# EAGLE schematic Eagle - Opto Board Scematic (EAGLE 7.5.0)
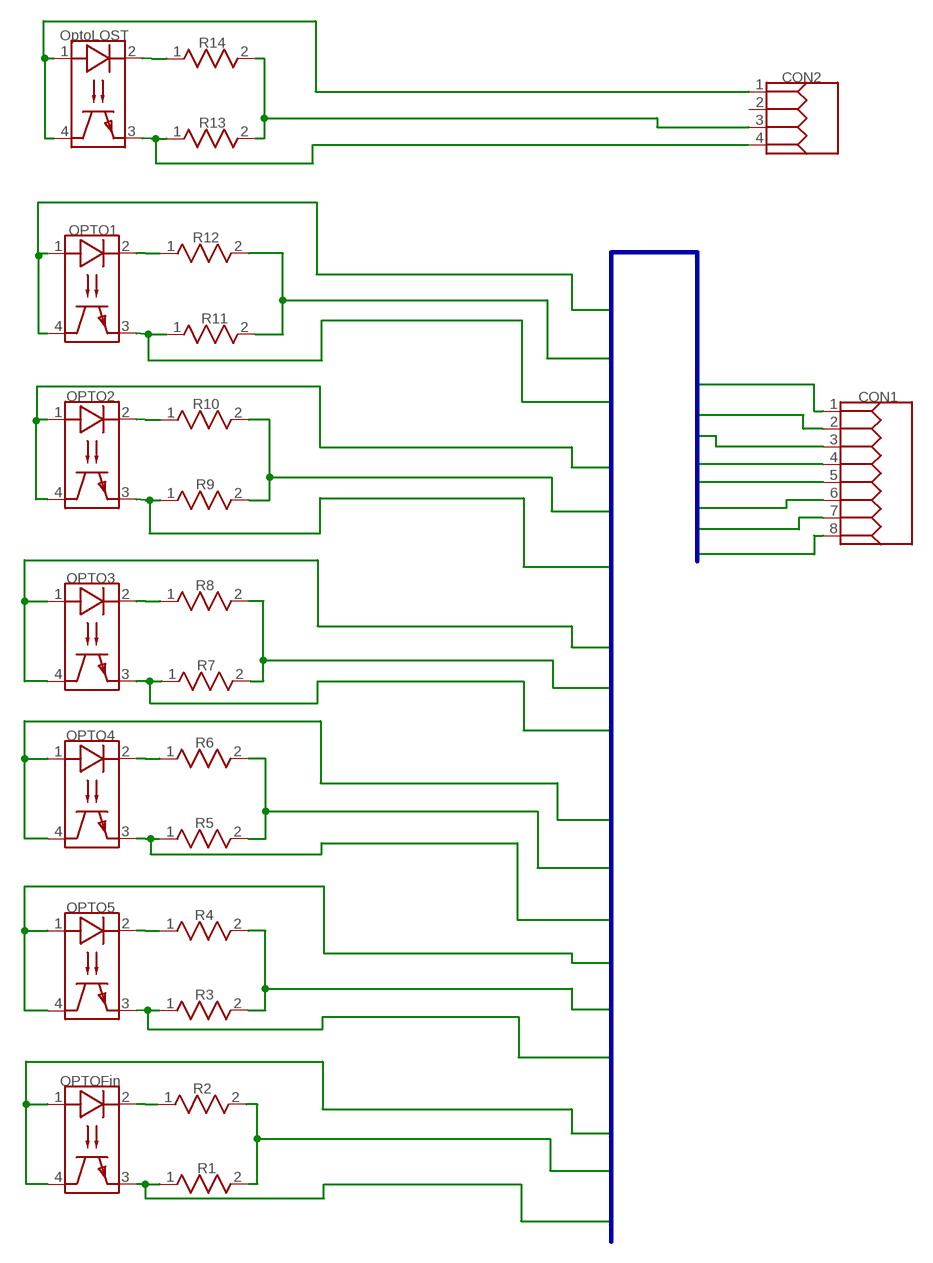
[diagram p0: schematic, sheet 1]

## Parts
CON1  51022-0800  [51022-0800]
CON2  51022-0400  [51022-0400]
OPTO1  TCRT1000  [TCRT1000]
OPTO2  TCRT1000  [TCRT1000]
OPTO3  TCRT1000  [TCRT1000]
OPTO4  TCRT1000  [TCRT1000]
OPTO5  TCRT1000  [TCRT1000]
OPTOFin  TCRT1000  [TCRT1000]
OptoLOST  TCRT1000  [TCRT1000]
R1  10K  RES  [RES_1206]
R2  150R  RES  [RES_1206]
R3  10K  RES  [RES_1206]
R4  150R  RES  [RES_1206]
R5  10K  RES  [RES_1206]
R6  150R  RES  [RES_1206]
R7  10K  RES  [RES_1206]
R8  150R  RES  [RES_1206]
R9  10K  RES  [RES_1206]
R10  150R  RES  [RES_1206]
R11  10K  RES  [RES_1206]
R12  150R  RES  [RES_1206]
R13  10K  RES  [RES_1206]
R14  150R  RES  [RES_1206]

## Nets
+5V: CON1.1 CON2.1 OPTO1.1(A) OPTO1.4(C) OPTO2.1(A) OPTO2.4(C) OPTO3.1(A) OPTO3.4(C) OPTO4.1(A) OPTO4.4(C) OPTO5.1(A) OPTO5.4(C) OPTOFin.1(A) OPTOFin.4(C) OptoLOST.1(A) OptoLOST.4(C)
GND: CON1.8 CON2.3 R1.2(B) R2.2(B) R3.2(B) R4.2(B) R5.2(B) R6.2(B) R7.2(B) R8.2(B) R9.2(B) R10.2(B) R11.2(B) R12.2(B) R13.2(B) R14.2(B)
Net_3: OPTO5.2(K) R4.1(A)
Net_32: OPTO1.2(K) R12.1(A)
Net_33: OPTO2.2(K) R10.1(A)
Net_34: OPTO3.2(K) R8.1(A)
Net_35: OPTO4.2(K) R6.1(A)
Net_37: OPTOFin.2(K) R2.1(A)
Net_39: OptoLOST.2(K) R14.1(A)
Opto1: CON1.2 OPTO1.3(E) R11.1(A)
Opto2: CON1.3 OPTO2.3(E) R9.1(A)
Opto3: CON1.4 OPTO3.3(E) R7.1(A)
Opto4: CON1.5 OPTO4.3(E) R5.1(A)
Opto5: CON1.6 OPTO5.3(E) R3.1(A)
OptoFIN: CON1.7 OPTOFin.3(E) R1.1(A)
OptoLOST: CON2.4 OptoLOST.3(E) R13.1(A)
Unconnected: CON2.2

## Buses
+5V,GND,Opto1,Opto2,Opto3,Opto4,Opto5,OptoFIN

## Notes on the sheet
- OptoLOST
- R14
- CON2
- R13
- OPTO1
- R12
- R11
- OPTO2 | CON1
- R10
- R9
- OPTO3
- R8
- R7
- OPTO4
- R6
- R5
- OPTO5
- R4
- R3
- OPTOFin
- R2
- R1

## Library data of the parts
CON1 = common:51022-0800; DATASHEET: http://datasheets.diptrace.com/con_board_in/510221400_sd.pdf; MANUFACTURER: Molex
CON2 = common:51022-0400; DATASHEET: http://datasheets.diptrace.com/con_board_in/510221400_sd.pdf; MANUFACTURER: Molex
OPTO1-OPTO5 OPTOFin OptoLOST = common:TCRT1000; DESCRIPTION: Optoisolator; UNTITLED: Opto Sensor
R1 R3 R5 R7 R9 R11 R13 = common:RES
R2 R4 R6 R8 R10 R12 R14 = common:RES; VALUE: 10K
